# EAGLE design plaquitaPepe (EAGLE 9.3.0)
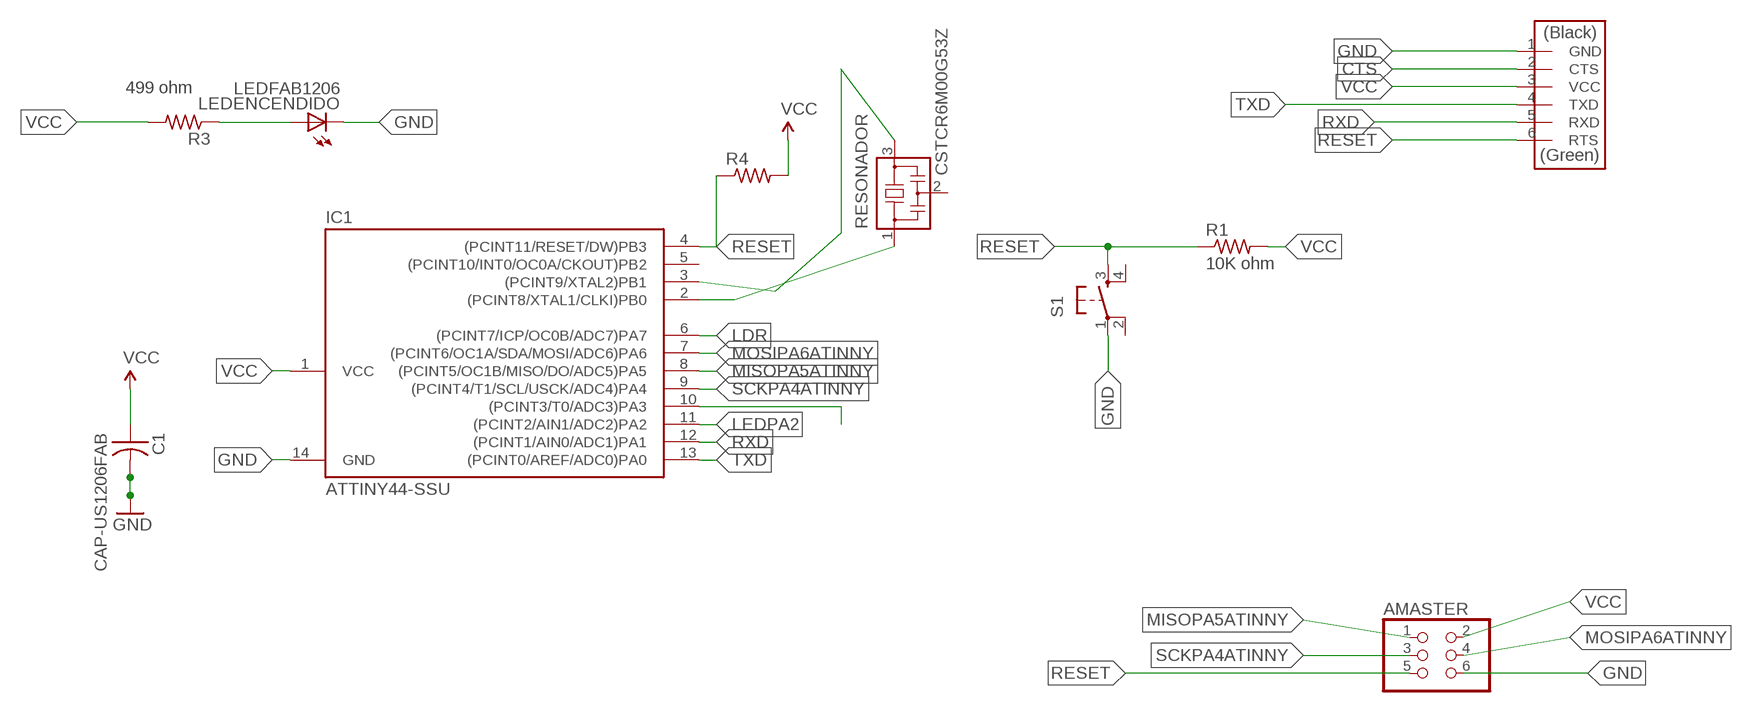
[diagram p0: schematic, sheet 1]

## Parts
AMASTER  PINHD-2X3-SMD  [2X03SMD]
C1  CAP-US1206FAB  [C1206FAB]
IC1  ATTINY44-SSU  [SOIC14]
J3  FTDI-SMD-HEADER  [1X06SMD]
LEDENCENDIDO  LEDFAB1206  [LED1206FAB]
R1  10K ohm  RES-US1206FAB  [R1206FAB]
R3  499 ohm  RES-US1206FAB  [R1206FAB]
R4  RES-US1206FAB  [R1206FAB]
RESONADOR  CSTCR6M00G53Z  [CSTCR6M]
S1  6MM_SWITCH6MM_SWITCH  [6MM_SWITCH]

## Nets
CTS: J3.2(CTS)
GND: AMASTER.6 C1.2 IC1.14(GND) J3.1(GND) LEDENCENDIDO.2(C) S1.1(P)
LDR: IC1.6((PCINT7/ICP/OC0B/ADC7)PA7)
LEDPA2: IC1.11((PCINT2/AIN1/ADC2)PA2)
MISOPA5ATINNY: AMASTER.1 IC1.8((PCINT5/OC1B/MISO/DO/ADC5)PA5)
MOSIPA6ATINNY: AMASTER.4 IC1.7((PCINT6/OC1A/SDA/MOSI/ADC6)PA6)
N$1: LEDENCENDIDO.1(A) R3.1
N$6: IC1.10((PCINT3/T0/ADC3)PA3)
RESET: AMASTER.5 IC1.4((PCINT11/RESET/DW)PB3) J3.6(RTS) R1.1 R4.1 S1.3(S)
RXD: IC1.12((PCINT1/AIN0/ADC1)PA1) J3.5(RXD)
SCKPA4ATINNY: AMASTER.3 IC1.9((PCINT4/T1/SCL/USCK/ADC4)PA4)
TXD: IC1.13((PCINT0/AREF/ADC0)PA0) J3.4(TXD)
VCC: AMASTER.2 C1.1 IC1.1(VCC) J3.3(VCC) R1.2 R3.2 R4.2
XTAL1: IC1.2((PCINT8/XTAL1/CLKI)PB0) RESONADOR.1
XTAL2: IC1.3((PCINT9/XTAL2)PB1) RESONADOR.3
Unconnected: IC1.5((PCINT10/INT0/OC0A/CKOUT)PB2) RESONADOR.2 S1.2(P1) S1.4(S1)

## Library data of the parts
AMASTER = fab:PINHD-2X3-SMD: PIN HEADER
C1 = fab:CAP-US
IC1 = fab:ATTINY44
J3 = fab:FTDI-SMD-HEADER
LEDENCENDIDO = fab:LED: LED
R1 R3 = fab:RES-US: Resistor (US Symbol)
R4 = 01_fab:RES-US: Resistor (US Symbol)
RESONADOR = murata-filter:CSTCR: Resonator Source: murata.co.jp; MPN: CSTCR6M00G53-R0; OC_FARNELL: 1170434; OC_NEWARK: 25M8759
S1 = fab:6MM_SWITCH: OMRON SWITCH

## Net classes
0 default: clearance 0.205 mm

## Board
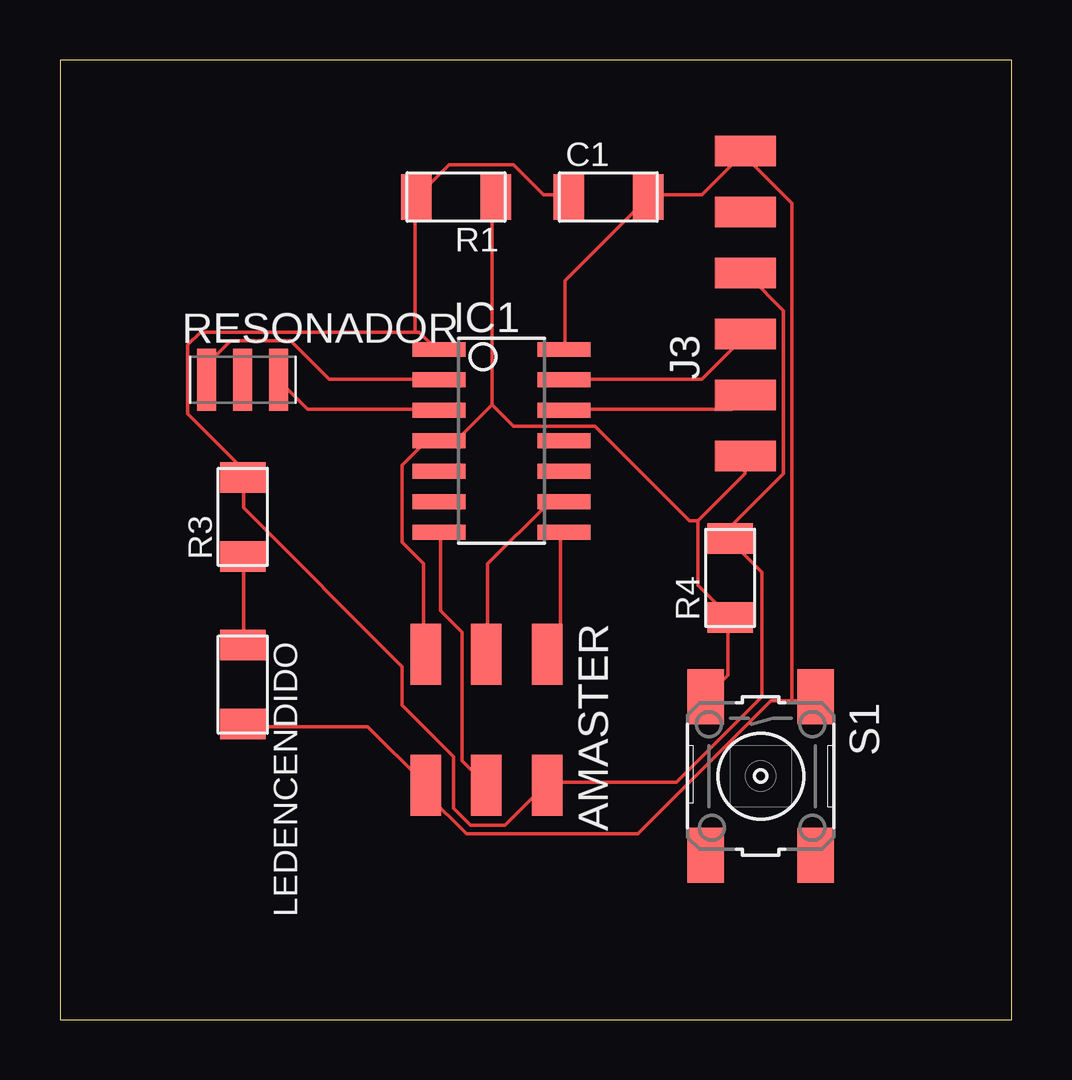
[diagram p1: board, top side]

Size 39.68 x 39.99 mm. Coordinates in mm from the lower left corner, seen from the top.
Outline: 0,0 39.68,0 39.68,39.99 0,39.99 0,0
Copper layers (1*16): Top 0.035mm / dielectric 1.5mm / Bottom 0.035mm
Design rules "default": minimum track width 6mil, minimum drill 0.35mm, track to track 6mil, track to pad 6mil, pad to pad 6mil, via to via 6mil, smd to smd 6mil, copper to edge 40mil, drill to drill 6mil, minimum pad ring 10mil, minimum via ring 8mil, stop-mask expansion 4mil, vias tented up to drill 0mil, thermal gap 10mil

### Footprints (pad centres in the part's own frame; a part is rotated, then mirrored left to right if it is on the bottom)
2X03SMD = smd 2.54 x 1.27: 1 -2.54,2.54; 2 2.92,2.54; 3 -2.54,0; 4 2.92,0; 5 -2.54,-2.54; 6 2.92,-2.54
C1206FAB = smd 1.27 x 1.905: 1 -1.651,0; 2 1.651,0
SOIC14 = smd 0.61 x 2.21: 1 -3.81,-2.603; 2 -2.54,-2.603; 3 -1.27,-2.603; 4 0,-2.603; 5 1.27,-2.603; 6 2.54,-2.603; 7 3.81,-2.603; 8 3.81,2.603; 9 2.54,2.603; 10 1.27,2.603; 11 0,2.603; 12 -1.27,2.603; 13 -2.54,2.603; 14 -3.81,2.603
1X06SMD = smd 2.54 x 1.27: 1 0,6.35; 2 0,3.81; 3 0,1.27; 4 0,-1.27; 5 0,-3.81; 6 0,-6.35
LED1206FAB = smd 1.27 x 1.905: 1 -1.651,0; 2 1.651,0
R1206FAB = smd 1.27 x 1.905: 1 -1.651,0; 2 1.651,0
CSTCR6M = smd 0.8 x 2.6: 1 -1.5,0; 2 0,0; 3 1.5,0
6MM_SWITCH = smd 2.286 x 1.524: 1 -3.302,2.286; 2 3.302,2.286; 3 -3.302,-2.286; 4 3.302,-2.286

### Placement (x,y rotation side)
AMASTER  17.78,12.7 270 top
C1  22.86,34.29 0 top
IC1  18.41,24.13 270 top
J3  28.57,29.84 0 top
LEDENCENDIDO  7.62,13.97 270 top
R1  16.51,34.29 180 top
R3  7.62,20.95 90 top
R4  27.94,18.41 90 top
RESONADOR  7.62,26.67 0 top
S1  29.21,10.16 270 top

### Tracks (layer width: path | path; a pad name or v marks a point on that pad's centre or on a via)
GND
  Top 0.152: IC1.14 21.05,27.95 21.05,30.8 24.45,34.2 C1.2 24.62,34.38 26.77,34.38 28.55,36.16 J3.1 28.73,36.16 28.73,35.81 30.52,34.02 30.52,13.29 | LEDENCENDIDO.2 7.65,12.22 12.83,12.22 15.15,9.9 AMASTER.6 15.33,9.72 15.33,9.36 16.94,7.75 24.09,7.75 29.63,13.29 30.52,13.29 | 30.52,13.29 31.41,13.29 S1.1
MISOPA5ATINNY
  Top 0.152: IC1.8 20.87,20.26 20.87,15.79 20.34,15.26 AMASTER.1
MOSIPA6ATINNY
  Top 0.152: IC1.7 15.87,20.26 15.87,17.04 16.76,16.15 16.76,10.79 17.65,9.9 AMASTER.4
N$1
  Top 0.152: LEDENCENDIDO.1 7.65,15.79 7.65,19.19 R3.1
RESET
  Top 0.152: S1.3 26.95,13.47 27.84,14.36 27.84,16.69 R4.1 27.84,16.86 26.59,18.12 26.59,20.8 | 26.59,20.8 28.55,22.76 28.55,23.48 J3.6 | 18.01,25.62 18.01,34.2 R1.1 | 18.01,25.62 16.58,24.19 15.87,24.19 IC1.4 15.69,24.01 15.15,24.01 14.26,23.12 14.26,19.9 15.15,19.01 15.15,15.26 AMASTER.5 | 26.59,20.8 26.23,20.8 22.3,24.73 18.91,24.73 18.01,25.62
RXD
  Top 0.152: IC1.12 21.05,25.44 28.02,25.44 28.55,25.98 J3.5
SCKPA4ATINNY
  Top 0.152: IC1.9 20.87,21.51 20.34,21.51 17.83,19.01 17.83,15.26 AMASTER.3
TXD
  Top 0.152: IC1.13 21.05,26.69 26.77,26.69 28.55,28.48 J3.4
VCC
  Top 0.152: 14.8,28.66 14.97,28.66 15.69,27.95 IC1.1 | 14.8,28.66 5.86,28.66 5.32,28.12 5.32,25.26 7.47,23.12 7.47,22.76 R3.2 7.65,22.58 7.65,21.33 14.26,14.72 14.26,13.11 16.4,10.97 16.4,8.82 17.12,8.11 18.55,8.11 20.16,9.72 AMASTER.2 20.34,9.9 25.7,9.9 29.27,13.47 29.27,18.65 28.02,19.9 R4.2 28.02,20.08 28.02,20.62 30.16,22.76 30.16,29.55 28.73,30.98 J3.3 | 14.8,28.66 14.8,34.2 R1.2 14.97,34.38 16.23,35.63 18.91,35.63 20.16,34.38 21.05,34.38 C1.1
XTAL1
  Top 0.152: IC1.2 15.69,26.69 11.22,26.69 9.61,28.3 7.11,28.3 6.22,27.41 6.22,26.69 RESONADOR.1
XTAL2
  Top 0.152: IC1.3 15.69,25.44 10.33,25.44 9.25,26.52 RESONADOR.3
